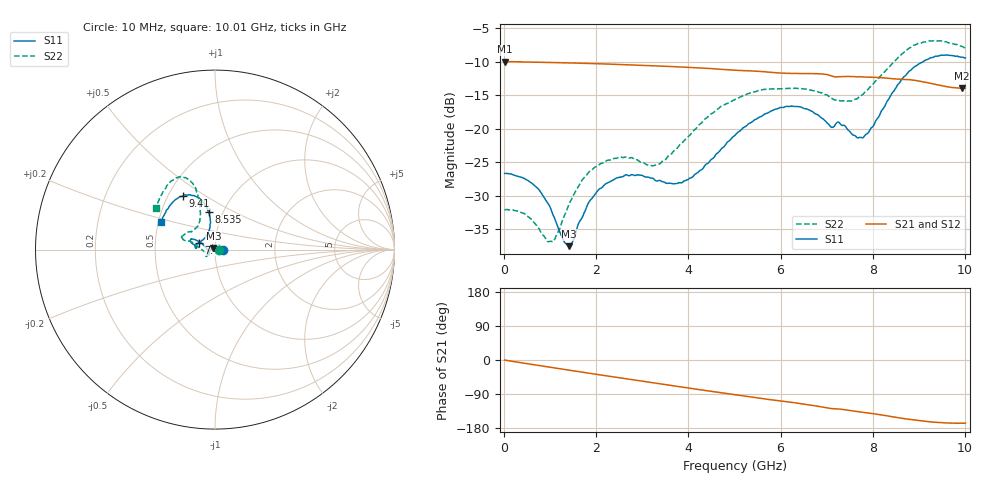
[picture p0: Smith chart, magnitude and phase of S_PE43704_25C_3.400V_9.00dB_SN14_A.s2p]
! Device ID: PE43704
! Dir: z:\PE43704\PE43704_Char_1_20130516\PE43704\AMB\3p400V\9p00dB
! Serial: 14
! Insertion: A
! Impedance: 50 ohm
! Temp: Amb
! VDD: 3.400V
! Attenuation Step: 9.00dB
! IDD: 1.140316e-01mA
#  Hz  S  RI  R  50
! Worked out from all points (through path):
!   401 points, 10 MHz to 10.01 GHz, reference 50 ohm
!   highest |S21| = -9.97 dB at 10 MHz (marker M1); lowest = -14.0 dB at 9.935 GHz (marker M2)
!   group delay of S21, straight-line fit = 48.1 ps
!   lowest |S11| = -37.5 dB at 1.41 GHz (marker M3), VSWR 1.03, Z = 49.1 + j0.948 ohm
!   |S11| at or under -10 dB: start of sweep to 9.091 GHz
!   |S22| runs from -36.9 to -6.8 dB; largest |S21 - S12| = 0.0025
!   S11 on the Smith chart (normalised r, x): 10 MHz: 1.10, +0.00; 7.46 GHz: 0.83, +0.06; 8.535 GHz: 0.86, +0.37; 9.41 GHz: 0.59, +0.40; 10.01 GHz: 0.52, +0.18
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1e7  0.0463 0.000276  0.3172 -0.00123  0.3173 -0.00114  0.0248 0.000311
6.1e8  0.0329 0.021  0.3076 -0.0642  0.3075 -0.0641  0.0127 0.0163
1.01e9  0.0127 0.0219  0.2949 -0.1032  0.2948 -0.1031  -0.00638 0.013
1.285e9  -0.00238 0.0146  0.2827 -0.1289  0.2828 -0.1287  -0.0213 0.00309
1.41e9  -0.00911 0.00966  0.2766 -0.1398  0.2766 -0.1399  -0.0273 -0.00256
1.685e9  -0.0214 -0.00145  0.2615 -0.1631  0.2615 -0.1631  -0.0378 -0.0162
2.01e9  -0.0308 -0.0137  0.241 -0.1881  0.241 -0.1879  -0.0431 -0.0295
2.41e9  -0.0345 -0.0246  0.2126 -0.2151  0.2128 -0.215  -0.0472 -0.0373
3.36e9  -0.0333 -0.0242  0.1353 -0.2608  0.1356 -0.2606  -0.0512 -0.0182
4.035e9  -0.0428 -0.00131  0.0755 -0.2762  0.0759 -0.2763  -0.0891 0.0113
5.01e9  -0.0805 0.0387  -0.00792 -0.2733  -0.00765 -0.2734  -0.1585 0.0477
5.935e9  -0.1283 0.0586  -0.0764 -0.2495  -0.0756 -0.2501  -0.1873 0.0647
6.685e9  -0.1299 0.036  -0.1277 -0.2239  -0.1281 -0.2237  -0.1757 0.0805
7.085e9  -0.1022 0.0168  -0.1525 -0.1965  -0.1535 -0.1973  -0.1376 0.0995
7.46e9  -0.0902 0.0386  -0.1659 -0.1811  -0.1656 -0.1814  -0.1046 0.1225
7.835e9  -0.0494 0.0747  -0.1832 -0.1601  -0.1834 -0.1605  -0.084 0.1687
8.36e9  -0.0264 0.1672  -0.2024 -0.1246  -0.2011 -0.1256  -0.0887 0.276
8.535e9  -0.0358 0.2084  -0.2072 -0.1108  -0.2059 -0.112  -0.1028 0.3202
8.91e9  -0.0796 0.2802  -0.2139 -0.0847  -0.213 -0.0834  -0.1525 0.3935
9.41e9  -0.1807 0.2976  -0.2051 -0.0555  -0.2053 -0.055  -0.2325 0.3881
9.935e9  -0.2877 0.1847  -0.195 -0.046  -0.196 -0.0458  -0.3201 0.2582
1.001e10  -0.2995 0.1551  -0.1954 -0.0463  -0.1965 -0.047  -0.3275 0.231
